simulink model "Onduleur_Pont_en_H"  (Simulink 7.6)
settings: Solver=ode15s  StartTime=0.0  StopTime=2  RelTol=1e-3
InitFcn:
  | clc
  | R=1e3; C=2500e-3/(5*pi);%1e-3/(5*pi)
  | 
  | R1=1e3
  | R2=R1;
StopFcn:
  | if 0
  | clc
  | close all, clc
  | load U_Umoy_charge.mat
  | plot(x(1,:),x(2,:),x(1,:),x(3,:))
  | xlabel('temps')
  | title('Tension charge et sa valeur moyenne')
  | grid
  | 
  | load I_Imoy_charge.mat
  | figure
  | plot(y(1,:),y(2,:),y(1,:),y(3,:))
  | xlabel('temps')
  | title('Courant charge et sa valeur moyenne')
  | grid
  | 
  | delete *.mat
  | end
libraries: fl_lib x24, nesl_utility x9, powerlib x8, elec_lib x4

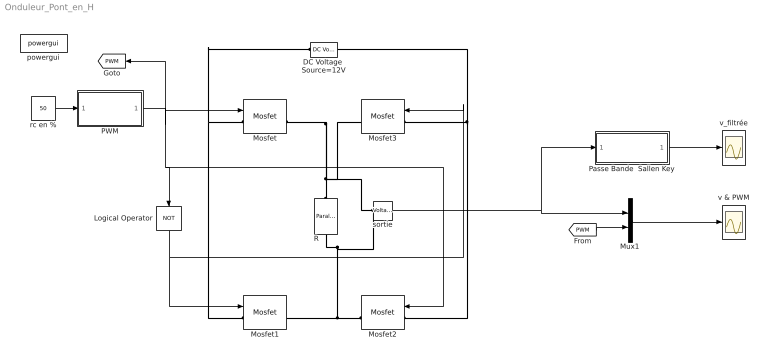
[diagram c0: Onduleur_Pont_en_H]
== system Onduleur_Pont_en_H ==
  DC Voltage  Source=12V : powerlib/Electrical Sources/DC Voltage Source  DialogController=POWERSYS.PowerSysDialog  SystemSampleTime=-1  Amplitude=12  Measurements=None
  Logical Operator : Logic  Operator=NOT  AllPortsSameDT=off  OutDataTypeStr=boolean
  Mosfet{,1..3} (4 alike) : powerlib/Power Electronics/Mosfet  DialogController=POWERSYS.PowerSysDialog  SystemSampleTime=-1  Ron=1e-6  Lon=0  Rd=0.001  Vfd=0  IC=0  Rs=1e8  Cs=inf  Measurements=on
  Mux1 : Mux  Inputs=2
  PWM : Subsystem
  Passe Bande  Sallen Key : Subsystem
  R : powerlib/Elements/Parallel RLC Branch  DialogController=POWERSYS.PowerSysDialog  PhysicalDomain=powersysdomain  SubClassName=unknown  LeftPortType=p1  RightPortType=p1  LConnTagsString=a  RConnTagsString=__new0  BranchType=R  Resistance=1e6  Inductance=1.0  SetiL0=off  InitialCurrent=0  Capacitance=25e-06  Setx0=off  InitialVoltage=0  Measurements=Branch voltage and current
  powergui : powerlib/powergui  SystemSampleTime=-1  SimulationMode=Continuous  SampleTime=0  frequency=60  SPID=off  DisableSnubberDevices=off  DisableRonSwitches=off  DisableVfSwitches=off  SwTol=0  Interpol=off  frequencyindice=0  echomessages=off  HookPort=off  DisplayEquations=off  FunctionMessages=off  EnableUseOfTLC=off  x0status=blocks  RestoreLinks=warning  ResistiveCurrentMeasurement=off  Frange=[0:2:500]  Ylog=off  Xlog=on  ShowGrid=off  save=off  variable=ZData  structure=v_filtree  ZoomFFT=off  StartTime=0.0  cycles=1  DisplayStyle=1  fundamental=60  FreqAxis=off  MaxFrequency=1000  frequencyindicesteady=1  RmsSteady=1  display=off  Ts=0  methode=off
  rc en % : Constant  Value=50
  sortie : powerlib/Measurements/Voltage Measurement  DialogController=POWERSYS.PowerSysDialog  SystemSampleTime=-1  PhasorSimulation=off  OutputType=Complex  PSBequivalent=0
  v & PWM : Scope
  v_filtrée : Scope
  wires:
  PWM/1(PWM) -> Mosfet/1, Logical Operator/1, Mosfet2/1, [PWM]
  rc en %/1 -> PWM/1(rc (%))
  Logical Operator/1 -> Mosfet1/1, Mosfet3/1
  Mux1/1 -> v & PWM/1
  [PWM] -> Mux1/2
  sortie/1 -> Mux1/1, Passe Bande  Sallen Key/1(e)
  Passe Bande  Sallen Key/1(s) -> v_filtrée/1
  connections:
  Mosfet2/RConn1 -- R/RConn1 -- sortie/LConn2 -- Mosfet1/RConn1
  Mosfet3/RConn1 -- Mosfet/RConn1 -- R/LConn1 -- sortie/LConn1
  Mosfet1/LConn1 -- DC Voltage  Source=12V/LConn1 -- Mosfet/LConn1
  Mosfet2/LConn1 -- Mosfet3/LConn1 -- DC Voltage  Source=12V/RConn1

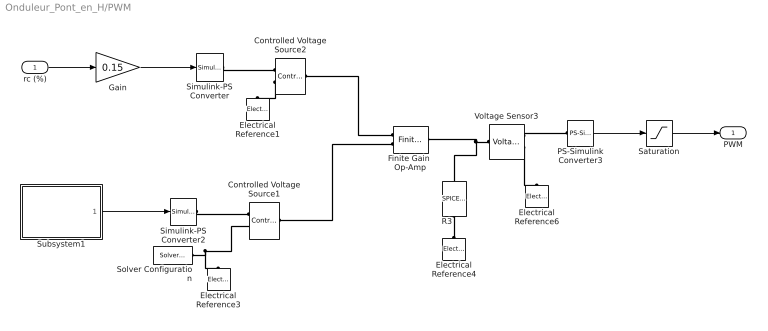
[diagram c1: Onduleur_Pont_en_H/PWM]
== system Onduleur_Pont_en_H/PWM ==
  rc (%) : Inport
  Controlled Voltage Source1 : fl_lib/Electrical/Electrical Sources/Controlled Voltage Source  DialogController=NetworkEngine.DynNeDlgSource  SystemSampleTime=-1  i_Log=off  v_Log=off  LocalVarNames=|current|voltage|power  LocalVarDescs=|Current (A)|Voltage (V)|Power (W)  LocalVarLogging=[0 0 0]
  Controlled Voltage Source2 : fl_lib/Electrical/Electrical Sources/Controlled Voltage Source  DialogController=NetworkEngine.DynNeDlgSource  SystemSampleTime=-1  i_Log=off  v_Log=off  LocalVarNames=|current|voltage|power  LocalVarDescs=|Current (A)|Voltage (V)|Power (W)  LocalVarLogging=[0 0 0]
  Electrical Reference{1,3..4,6} (4 alike) : fl_lib/Electrical/Electrical Elements/Electrical Reference  DialogController=NetworkEngine.DynNeDlgSource  SystemSampleTime=-1  i_Log=off  LocalVarNames=|i  LocalVarDescs=|i  LocalVarLogging=[]
  Finite Gain  Op-Amp : elec_lib/Integrated Circuits/Finite Gain Op-Amp  DialogController=NetworkEngine.DynNeDlgSource  SystemSampleTime=-1  A=1000  Rin=1e+06 Ohm  Rout=100 Ohm  Vmin=-12 V  Vmax=12 V  LocalVarNames=|power  LocalVarDescs=|Dissipated power (W)  LocalVarLogging=0
  Gain : Gain  Gain=0.15
  PS-Simulink Converter3 : nesl_utility/PS-Simulink Converter  DialogController=NetworkEngine.DynNeUtilDlgSource  SystemSampleTime=-1  PhysicalDomain=network_engine_domain  LeftPortType=input  RightPortType=output  SubClassName=ps_output  Unit=1  AffineConversion=off
  R3 : elec_lib/Additional Components/SPICE-Compatible Components/Passive Devices/SPICE Resistor  DialogController=NetworkEngine.DynNeDlgSource  SystemSampleTime=-1  SCALE=1  R_param=1  R=10e3 Ohm  RSH=0 Ohm  LENGTH=1e-06 m  WIDTH=1e-06 m  NARROW=0 m  T_param=1  TC1=0 1/K  TC2=0 1/K^2  TOFFSET=0 K  TFIXED=300.15 K  TMEAS=300.15 K  LocalVarLogging=[]
  Saturation : Saturate  UpperLimit=1  LowerLimit=0
  Simulink-PS Converter : nesl_utility/Simulink-PS Converter  DialogController=NetworkEngine.DynNeUtilDlgSource  SystemSampleTime=-1  PhysicalDomain=network_engine_domain  LeftPortType=input  RightPortType=output  SubClassName=ps_input  Unit=1  AffineConversion=off  InputFilterTimeConstant=.001  UdotUserProvided=0
  Simulink-PS Converter2 : nesl_utility/Simulink-PS Converter  DialogController=NetworkEngine.DynNeUtilDlgSource  SystemSampleTime=-1  PhysicalDomain=network_engine_domain  LeftPortType=input  RightPortType=output  SubClassName=ps_input  Unit=1  AffineConversion=off  InputFilterTimeConstant=.001  UdotUserProvided=0
  Solver Configuration : nesl_utility/Solver Configuration  DialogController=NetworkEngine.DynNeUtilDlgSource  SystemSampleTime=-1  PhysicalDomain=network_engine_domain  LeftPortType=input  RightPortType=generic  SubClassName=solver  Accelerate=off  Profile=off  ResidualTolerance=1e-12  MaxNonlinIter=12  MaxModeIter=2  DoFixedCost=on  UseLocalSampling=off  DoDC=off  LinearAlgebra=Sparse  LocalSolverSampleTime=.001  LocalSolverChoice=NE_BACKWARD_EULER_ADVANCER  UseLocalSolver=off
  Subsystem1 : Subsystem
  Voltage Sensor3 : fl_lib/Electrical/Electrical Sensors/Voltage Sensor  DialogController=NetworkEngine.DynNeDlgSource  SystemSampleTime=-1  i1_Log=off  v1_Log=off  LocalVarNames=|i1|v1  LocalVarDescs=|i1|v1  LocalVarLogging=[]
  PWM : Outport
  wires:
  Gain/1 -> Simulink-PS Converter/1
  Saturation/1 -> PWM/1
  PS-Simulink Converter3/1 -> Saturation/1
  rc (%)/1 -> Gain/1
  Subsystem1/1(tri) -> Simulink-PS Converter2/1
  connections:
  Voltage Sensor3/RConn1 -- PS-Simulink Converter3/LConn1
  Voltage Sensor3/LConn1 -- R3/RConn1 -- Finite Gain  Op-Amp/RConn1
  Voltage Sensor3/RConn2 -- Electrical Reference6/LConn1
  Electrical Reference4/LConn1 -- R3/LConn1
  Controlled Voltage Source2/RConn2 -- Electrical Reference1/LConn1
  Simulink-PS Converter/RConn1 -- Controlled Voltage Source2/RConn1
  Finite Gain  Op-Amp/LConn1 -- Controlled Voltage Source2/LConn1
  Solver Configuration/RConn1 -- Electrical Reference3/LConn1 -- Controlled Voltage Source1/RConn2
  Simulink-PS Converter2/RConn1 -- Controlled Voltage Source1/RConn1
  Controlled Voltage Source1/LConn1 -- Finite Gain  Op-Amp/LConn2

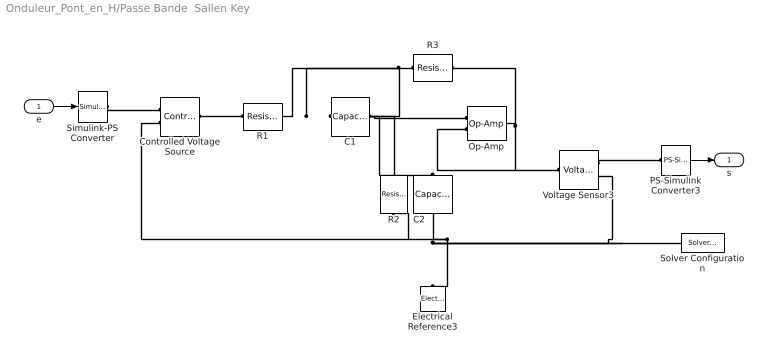
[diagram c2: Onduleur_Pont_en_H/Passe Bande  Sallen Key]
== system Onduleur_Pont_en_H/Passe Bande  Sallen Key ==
  e : Inport
  C1 : fl_lib/Electrical/Electrical Elements/Capacitor  DialogController=NetworkEngine.DynNeDlgSource  SystemSampleTime=-1  c=C uF  v0=0 V  r=1e-6 Ohm  g=0 1/Ohm  i_Log=off  v_Log=off  vc_Log=off  LocalVarNames=|i|v|vc  LocalVarDescs=|i|v|Internal variable for voltage across capacitor term  LocalVarLogging=[0 0 0]
  C2 : fl_lib/Electrical/Electrical Elements/Capacitor  DialogController=NetworkEngine.DynNeDlgSource  SystemSampleTime=-1  c=C uF  v0=0 V  r=1e-6 Ohm  g=0 1/Ohm  i_Log=off  v_Log=off  vc_Log=off  LocalVarNames=|i|v|vc  LocalVarDescs=|i|v|Internal variable for voltage across capacitor term  LocalVarLogging=[0 0 0]
  Controlled Voltage Source : fl_lib/Electrical/Electrical Sources/Controlled Voltage Source  DialogController=NetworkEngine.DynNeDlgSource  SystemSampleTime=-1  i_Log=off  v_Log=off  LocalVarNames=|i|v  LocalVarDescs=|i|v  LocalVarLogging=[0 0]
  Electrical Reference3 : fl_lib/Electrical/Electrical Elements/Electrical Reference  DialogController=NetworkEngine.DynNeDlgSource  SystemSampleTime=-1  i_Log=off  LocalVarNames=|i  LocalVarDescs=|i  LocalVarLogging=[]
  Op-Amp : fl_lib/Electrical/Electrical Elements/Op-Amp  DialogController=NetworkEngine.DynNeDlgSource  SystemSampleTime=-1  i1_Log=off  v1_Log=off  outI_Log=off  LocalVarNames=|i1|v1|outI  LocalVarDescs=|i1|v1|outI  LocalVarLogging=[]
  PS-Simulink Converter3 : nesl_utility/PS-Simulink Converter  DialogController=NetworkEngine.DynNeUtilDlgSource  SystemSampleTime=-1  PhysicalDomain=network_engine_domain  LeftPortType=input  RightPortType=output  SubClassName=ps_output  Unit=1  AffineConversion=off
  R1 : fl_lib/Electrical/Electrical Elements/Resistor  DialogController=NetworkEngine.DynNeDlgSource  SystemSampleTime=-1  R=R kOhm  i_Log=off  v_Log=off  LocalVarNames=|current|voltage|power  LocalVarDescs=|Resistor current (A)|Voltage across resistor (V)|Power (W)  LocalVarLogging=[0 0 0]
  R2 : fl_lib/Electrical/Electrical Elements/Resistor  DialogController=NetworkEngine.DynNeDlgSource  SystemSampleTime=-1  R=R kOhm  i_Log=off  v_Log=off  LocalVarNames=|current|voltage|power  LocalVarDescs=|Resistor current (A)|Voltage across resistor (V)|Power (W)  LocalVarLogging=[0 0 0]
  R3 : fl_lib/Electrical/Electrical Elements/Resistor  DialogController=NetworkEngine.DynNeDlgSource  SystemSampleTime=-1  R=R kOhm  i_Log=off  v_Log=off  LocalVarNames=|current|voltage|power  LocalVarDescs=|Resistor current (A)|Voltage across resistor (V)|Power (W)  LocalVarLogging=[0 0 0]
  Simulink-PS Converter : nesl_utility/Simulink-PS Converter  DialogController=NetworkEngine.DynNeUtilDlgSource  SystemSampleTime=-1  PhysicalDomain=network_engine_domain  LeftPortType=input  RightPortType=output  SubClassName=ps_input  Unit=1  AffineConversion=off  InputFilterTimeConstant=.001  UdotUserProvided=0
  Solver Configuration : nesl_utility/Solver Configuration  DialogController=NetworkEngine.DynNeUtilDlgSource  SystemSampleTime=-1  PhysicalDomain=network_engine_domain  LeftPortType=input  RightPortType=generic  SubClassName=solver  Accelerate=off  Profile=off  ResidualTolerance=1e-9  MaxNonlinIter=12  MaxModeIter=2  DoFixedCost=off  UseLocalSampling=off  DoDC=off  LinearAlgebra=Sparse  LocalSolverSampleTime=.001  LocalSolverChoice=NE_BACKWARD_EULER_ADVANCER  UseLocalSolver=off
  Voltage Sensor3 : fl_lib/Electrical/Electrical Sensors/Voltage Sensor  DialogController=NetworkEngine.DynNeDlgSource  SystemSampleTime=-1  i1_Log=off  v1_Log=off  LocalVarNames=|i1|v1  LocalVarDescs=|i1|v1  LocalVarLogging=[]
  s : Outport
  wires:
  PS-Simulink Converter3/1 -> s/1
  e/1 -> Simulink-PS Converter/1
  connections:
  Voltage Sensor3/RConn1 -- PS-Simulink Converter3/LConn1
  Simulink-PS Converter/RConn1 -- Controlled Voltage Source/RConn1
  Controlled Voltage Source/LConn1 -- R1/LConn1
  Controlled Voltage Source/RConn2 -- Electrical Reference3/LConn1 -- C2/RConn1 -- Solver Configuration/RConn1 -- Voltage Sensor3/RConn2 -- R2/LConn1
  C1/LConn1 -- C2/LConn1 -- Op-Amp/LConn1 -- R2/RConn1
  R3/RConn1 -- Op-Amp/RConn1 -- Voltage Sensor3/LConn1 -- Op-Amp/LConn2
  R3/LConn1 -- R1/RConn1 -- C1/RConn1

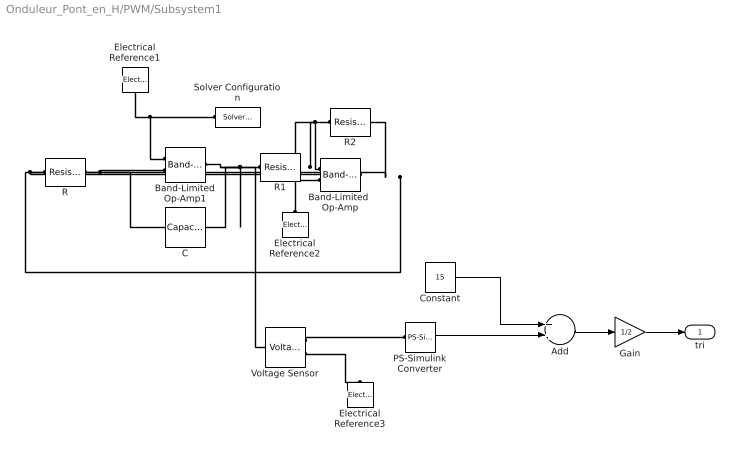
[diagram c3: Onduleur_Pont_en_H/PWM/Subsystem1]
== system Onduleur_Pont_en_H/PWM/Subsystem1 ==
  Add : Sum
  Band-Limited  Op-Amp : elec_lib/Integrated Circuits/Band-Limited Op-Amp  DialogController=NetworkEngine.DynNeDlgSource  SystemSampleTime=-1  A=1000  Rin=1e+06 Ohm  Rout=100 Ohm  Vmin=-15 V  Vmax=15 V  Vdotmax=1000 V/s  f=1e+05 Hz  V0=0 V  LocalVarNames=|power  LocalVarDescs=|Dissipated power (W)  LocalVarLogging=0
  Band-Limited Op-Amp1 : elec_lib/Integrated Circuits/Band-Limited Op-Amp  DialogController=NetworkEngine.DynNeDlgSource  SystemSampleTime=-1  A=1000  Rin=1e+06 Ohm  Rout=100 Ohm  Vmin=-15 V  Vmax=15 V  Vdotmax=1000 V/s  f=1e+05 Hz  V0=0 V  LocalVarNames=|power  LocalVarDescs=|Dissipated power (W)  LocalVarLogging=0
  C : fl_lib/Electrical/Electrical Elements/Capacitor  DialogController=NetworkEngine.DynNeDlgSource  SystemSampleTime=-1  c=0.5e-4 F  v0=0.1 V  r=1e-6 Ohm  g=0 1/Ohm  i_Log=off  v_Log=off  vc_Log=off  LocalVarNames=|current|voltage|power  LocalVarDescs=|Capacitor current (A)|Voltage across capacitor (V)|Power (W)  LocalVarLogging=[0 0 0]
  Constant : Constant  Value=15
  Electrical Reference1 : fl_lib/Electrical/Electrical Elements/Electrical Reference  DialogController=NetworkEngine.DynNeDlgSource  SystemSampleTime=-1  i_Log=off  LocalVarNames=|i  LocalVarDescs=|i  LocalVarLogging=[]
  Electrical Reference2 : fl_lib/Electrical/Electrical Elements/Electrical Reference  DialogController=NetworkEngine.DynNeDlgSource  SystemSampleTime=-1  i_Log=off  LocalVarNames=|i  LocalVarDescs=|i  LocalVarLogging=[]
  Electrical Reference3 : fl_lib/Electrical/Electrical Elements/Electrical Reference  DialogController=NetworkEngine.DynNeDlgSource  SystemSampleTime=-1  i_Log=off  LocalVarNames=|i  LocalVarDescs=|i  LocalVarLogging=[]
  Gain : Gain  Gain=1/2
  PS-Simulink Converter : nesl_utility/PS-Simulink Converter  DialogController=NetworkEngine.DynNeUtilDlgSource  SystemSampleTime=-1  PhysicalDomain=network_engine_domain  LeftPortType=input  RightPortType=output  SubClassName=ps_output  Unit=1  AffineConversion=off
  R : fl_lib/Electrical/Electrical Elements/Resistor  DialogController=NetworkEngine.DynNeDlgSource  SystemSampleTime=-1  R=1000 Ohm  i_Log=off  v_Log=off  LocalVarNames=|current|voltage|power  LocalVarDescs=|Resistor current (A)|Voltage across resistor (V)|Power (W)  LocalVarLogging=[0 0 0]
  R1 : fl_lib/Electrical/Electrical Elements/Resistor  DialogController=NetworkEngine.DynNeDlgSource  SystemSampleTime=-1  R=10e3 Ohm  i_Log=off  v_Log=off  LocalVarNames=|current|voltage|power  LocalVarDescs=|Resistor current (A)|Voltage across resistor (V)|Power (W)  LocalVarLogging=[0 0 0]
  R2 : fl_lib/Electrical/Electrical Elements/Resistor  DialogController=NetworkEngine.DynNeDlgSource  SystemSampleTime=-1  R=10e3 Ohm  i_Log=off  v_Log=off  LocalVarNames=|current|voltage|power  LocalVarDescs=|Resistor current (A)|Voltage across resistor (V)|Power (W)  LocalVarLogging=[0 0 0]
  Solver Configuration : nesl_utility/Solver Configuration  DialogController=NetworkEngine.DynNeUtilDlgSource  SystemSampleTime=-1  PhysicalDomain=network_engine_domain  LeftPortType=input  RightPortType=generic  SubClassName=solver  Accelerate=off  Profile=off  ResidualTolerance=1e-9  MaxNonlinIter=12  MaxModeIter=2  DoFixedCost=off  UseLocalSampling=off  DoDC=off  LinearAlgebra=Sparse  LocalSolverSampleTime=.001  LocalSolverChoice=NE_BACKWARD_EULER_ADVANCER  UseLocalSolver=off
  Voltage Sensor : fl_lib/Electrical/Electrical Sensors/Voltage Sensor  DialogController=NetworkEngine.DynNeDlgSource  SystemSampleTime=-1  i1_Log=off  v1_Log=off  LocalVarNames=|i1|v1  LocalVarDescs=|i1|v1  LocalVarLogging=[]
  tri : Outport
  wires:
  PS-Simulink Converter/1 -> Add/2
  Constant/1 -> Add/1
  Add/1 -> Gain/1
  Gain/1 -> tri/1
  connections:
  Voltage Sensor/RConn1 -- PS-Simulink Converter/LConn1
  Band-Limited Op-Amp1/RConn1 -- R1/LConn1 -- C/RConn1 -- Voltage Sensor/LConn1
  R/RConn1 -- C/LConn1 -- Band-Limited Op-Amp1/LConn2
  Solver Configuration/RConn1 -- Band-Limited Op-Amp1/LConn1 -- Electrical Reference1/LConn1
  R/LConn1 -- Band-Limited  Op-Amp/RConn1 -- R2/RConn1
  Electrical Reference2/LConn1 -- Band-Limited  Op-Amp/LConn2
  R2/LConn1 -- Band-Limited  Op-Amp/LConn1 -- R1/RConn1
  Voltage Sensor/RConn2 -- Electrical Reference3/LConn1
